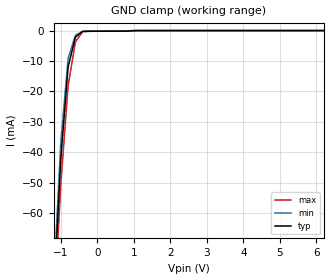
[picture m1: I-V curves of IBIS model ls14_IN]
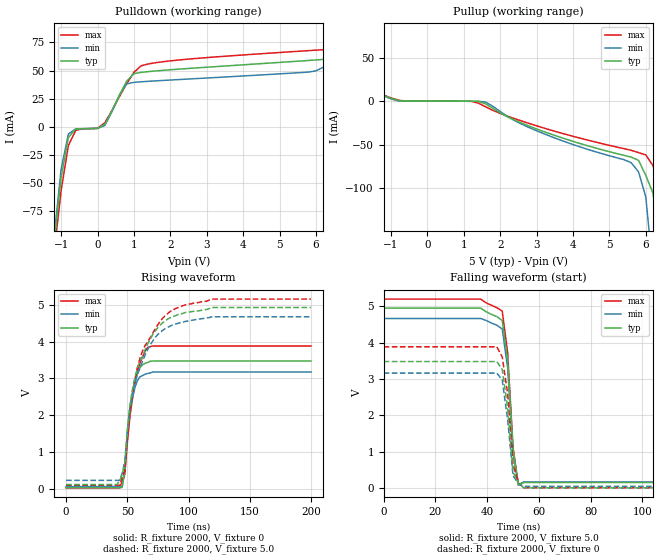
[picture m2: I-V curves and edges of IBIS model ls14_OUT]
|   TEXAS INSTRUMENTS INCORPORATED
|   Standard Linear and Logic Group
|   IBIS Model of SN74LS14
|   HEX SCHMITT- TRIGGER INVERTERS
|   SOIC 14-pin (D), SSOP 14-pin (DB),PDIP 14-pin (N)
[IBIS Ver]   3.2
[Comment Char]  |_char
[File Name]   sn74ls14.ibs
[File Rev]   3.2 | a_die
[Date]   11/12/04
[Source]   File originated at Texas Instruments, Inc.
[Notes]   The following is a sample IBIS file for the LS14.
   - FILE REV HISTORY
   - 3.2 Re-Release IBIS file on 11/16/04
   - Power clamp data deleted as there is no power-clamp diode.
   - All test data contained in this file are derived from
   actual measurement.
   - The measurement used NS package.
   - We have data across voltage and temperature, but not
   across process.
   - File created by Nobuhisa Ohtsubo, SLL Product Engineering.
[Disclaimer] Property of Texas Instruments Incorporated.  Unauthorized
   reproduction and/or distribution is strictly prohibited.
   This product is protected under copyright law.
   Created 2000, (C) Copyright 2000, Texas Instruments Inc.,
   All Rights Reserved.
   UNLESS THERE IS A SIGNED, WRITTEN AGREEMENT TO THE
   CONTRARY, TEXAS INSTRUMENTS () IS PROVIDING THE IBIS
   MODELS  AND WITHOUT ANY WARRANTY, EXPRESSED OR
   IMPLIED.  TI assumes no liability for:
   1) the accuracy of the IBIS models provided to your
   company;
   2) the proper functioning of these IBIS Models in your
   design or for any resulting applications; or
   3) infringement of patents, copyrights or intellectual
   property rights resulting from your use of these IBIS
   models.
   TI provides IBIS Models as a service to our customers.
   You and your company shall not distribute, sell or give
   these models to anyone else without prior written
   permission from TI.
   TI reserves the right to make changes to our products or
   to discontinue any semiconductor product or service
   without notice, and advises our customers to obtain the
   latest version of relevant information to verify, before
   placing orders, that the information being relied on is
   current.
   Please be aware that your receipt and use of the IBIS
   information provided shall serve as acceptance of these
   terms and conditions.  If you do not accept these terms,
   you should return or destroy the IBIS models and any
   other accompanying information immediately.
|   Component ls14_D
[Component]   ls14_D
[Manufacturer]  Texas Instruments, Inc.
[Package]
|   typ   min   max
R_pkg   0.031   0.028   0.034
L_pkg   3.109nH   2.462nH   3.889nH
C_pkg   0.473pF   0.363pF   0.628pF
[Pin]   signal_name   model_name   R_pin   L_pin   C_pin
1   1A   ls14_IN   0.033   3.854nH   0.622pF
2   1Y   ls14_OUT   0.032   3.188nH   0.473pF
3   2A   ls14_IN   0.028   2.462nH   0.377pF
4   2Y   ls14_OUT   0.031   2.596nH   0.363pF
5   3A   ls14_IN   0.028   2.521nH   0.372pF
6   3Y   ls14_OUT   0.034   3.250nH   0.476pF
7   GND   GND   0.034   3.889nH   0.628pF
8   4Y   ls14_IN   0.034   3.889nH   0.628pF
9   4A   ls14_OUT   0.034   3.250nH   0.476pF
10   5Y   ls14_IN   0.028   2.521nH   0.372pF
11   5A   ls14_OUT   0.031   2.596nH   0.364pF
12   6Y   ls14_IN   0.028   2.462nH   0.377pF
13   6A   ls14_OUT   0.032   3.188nH   0.473pF
14   VCC   POWER   0.033   3.854nH   0.622pF
| Component ls14_NS 14-pin SOP
[Component]   ls14_NS
[Manufacturer]   Texas Instruments, Inc.
[Package]
|   typ   min   max
R_pkg   0.045   0.039   0.054
L_pkg   3.796nH   2.561nH   4.952nH
C_pkg   0.528pF   0.288pF   0.710pF
[Pin]   signal_name   model_name   R_pin   L_pin   C_pin
1   1A   ls14_IN   0.047   4.867nH   0.706pF
2   1Y   ls14_OUT   0.051   4.083nH   0.592pF
3   2A   ls14_IN   0.041   2.915nH   0.376pF
4   2Y   ls14_OUT   0.039   2.561nH   0.288pF
5   3A   ls14_IN   0.041   3.101nH   0.430pF
6   3Y   ls14_OUT   0.047   4.047nH   0.589pF
7   GND   GND   0.051   4.909nH   0.700pF
8   4Y   ls14_IN   0.045   4.784nH   0.694pF
9   4A   ls14_OUT   0.054   4.176nH   0.597pF
10   5Y   ls14_IN   0.039   3.287nH   0.449pF
11   5A   ls14_OUT   0.039   2.586nH   0.294pF
12   6Y   ls14_IN   0.040   2.802nH   0.371pF
13   6A   ls14_OUT   0.049   4.080nH   0.593pF
14   VCC   POWER   0.052   4.952nH   0.710pF
| Component ls14_N 14-pin PDIP
[Component]   ls14_N
[Manufacturer]   Texas Instruments, Inc.
[Package]
|   typ   min   max
R_pkg   4.500e-02   3.700e-02   6.300e-02
L_pkg   5.407e-09   3.922e-09   6.942e-09
C_pkg   3.890e-13   2.050e-13   6.040e-13
[Pin]   signal_name   model_name   R_pin   L_pin   C_pin
1   1A   ls14_IN   6.300e-02   6.942e-09   6.040e-13
2   1Y   ls14_OUT   3.700e-02   6.200e-09   4.060e-13
3   2A   ls14_IN   4.200e-02   4.389e-09   3.220e-13
4   2Y   ls14_OUT   3.800e-02   3.922e-09   2.050e-13
5   3A   ls14_IN   3.900e-02   4.301e-09   2.980e-13
6   3Y   ls14_OUT   3.800e-02   5.329e-09   3.560e-13
7   GND   GND   5.300e-02   6.510e-09   5.440e-13
8   4Y   ls14_OUT   5.300e-02   6.437e-09   5.390e-13
9   4A   ls14_IN   3.900e-02   5.352e-09   3.470e-13
10   5Y   ls14_OUT   4.200e-02   4.473e-09   2.970e-13
11   5A   ls14_IN   4.400e-02   4.326e-09   2.250e-13
12   6Y   ls14_OUT   4.200e-02   4.295e-09   2.800e-13
13   6A   ls14_IN   4.200e-02   6.318e-09   4.180e-13
14   VCC   POWER   6.100e-02   6.900e-09   6.030e-13
|   Component ls14_DB
[Component]   ls14_DB
[Manufacturer]  Texas Instruments, Inc.
[Package]
|   typ   min   max
R_pkg   0.044   0.041   0.046
L_pkg   3.551nH   3.258nH   3.927nH
C_pkg   0.402pF   0.360pF   0.421pF
[Pin]   signal_name   model_name   R_pin   L_pin   C_pin
1   1A   ls14_IN   0.046   3.927nH   0.408pF
2   1Y   ls14_OUT   0.044   3.587nH   0.421pF
3   2A   ls14_IN   0.041   3.289nH   0.398pF
4   2Y   ls14_OUT   0.042   3.258nH   0.360pF
5   3A   ls14_IN   0.041   3.286nH   0.403pF
6   3Y   ls14_OUT   0.044   3.586nH   0.421pF
7   GND   GND   0.046   3.927nH   0.408pF
8   4Y   ls14_IN   0.046   3.927nH   0.408pF
9   4A   ls14_OUT   0.044   3.586nH   0.421pF
10   5Y   ls14_IN   0.041   3.286nH   0.403pF
11   5A   ls14_OUT   0.043   3.258nH   0.360pF
12   6Y   ls14_IN   0.041   3.289nH   0.398pF
13   6A   ls14_OUT   0.044   3.587nH   0.421pF
14   VCC   POWER   0.046   3.927nH   0.408pF
| Models and submodels in the file (2): ls14_IN (Input), ls14_OUT (Output)
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|   Model ls14_IN
[Model]   ls14_IN
Model_type  Input
Polarity   Inverting
Vinl = 0.8
Vinh = 2.0
| variable   typ   min   max
C_comp   1.33pf   1.00pf   1.66pf
[Temperature Range]   25   0   70
[Voltage Range]   5.0   4.75   5.25
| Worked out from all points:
|   GND clamp passes 1 mA (typ) near -0.48 V on its own axis
[GND Clamp]
|   Voltage   I(typ)   I(min)   I(max)
-5V       -1.315A    -1.382A    -1.195A
-1.2V     -88.77mA   -83.57mA   -95.34mA
-1V       -42.05mA   -36.6mA    -50.6mA
-800mV    -11.89mA   -9.112mA   -18.14mA
-600mV    -2.169mA   -1.53mA    -3.706mA
-400mV    -247.6uA   -246.4uA   -364uA
1.2V      -366.4nA   -227.1nA   -428nA
10V       15.2nA     25.25nA    57.62nA
|   Model ls14_OUT
[Model]   ls14_OUT
Model_type  Output
Polarity   Inverting
Vmeas = 1.3v
Cref = 15pf
Rref = 2000
Vref = 0V
| variable   typ   min   max
C_comp   5.8pf   4.35pf   7.25pf
[Temperature Range]   25   0   70
[Voltage Range]   5.0   4.75   5.25
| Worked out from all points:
|   slope of the pulldown table from 0 to 0.75 V, typ, clamps not added: 19.3 ohm
|   slope of the pullup table from 0 to 0.75 V, typ, clamps not added: 31.3 kohm
|   rising waveform, R_fixture 2000, V_fixture 0: 20-80 % time 7.12ns typ, 6.52ns min, 8.96ns max; typ from 0.022 V to 3.47 V
|   falling waveform, R_fixture 2000, V_fixture 5.0: 20-80 % time 2.91ns typ, 2.91ns min, 2.89ns max; typ from 4.95 V to 0.156 V
|   rising waveform, R_fixture 2000, V_fixture 5.0: 20-80 % time 18.3ns typ, 17.7ns min, 19.9ns max; typ from 0.11 V to 4.93 V
|   falling waveform, R_fixture 2000, V_fixture 0: 20-80 % time 2.93ns typ, 2.89ns min, 3.01ns max; typ from 3.48 V to 0.011 V
[Pulldown]
|   Voltage   I(typ)   I(min)   I(max)
-5V       -1.637A    -1.754A    -1.459A
-1.2V     -106.1mA   -99.87mA   -113.9mA
-1V       -45.11mA   -37.62mA   -56.62mA
-800mV    -9.35mA    -6.287mA   -16.52mA
-600mV    -1.967mA   -1.716mA   -3.114mA
200mV     2.325mA    1.242mA    3.681mA
800mV     40.65mA    38.22mA    38.31mA
1.2V      48.39mA    40.06mA    54.31mA
6V        59.43mA    49.77mA    68.14mA
6.6V      64.1mA     61.17mA    69.39mA
7.8V      87.38mA    87.2mA     82.72mA
10V       130.7mA    135.2mA    111.3mA
[Pullup]
|   Voltage   I(typ)   I(min)   I(max)
-5V       79.98mA    83.78mA    71.9mA
-1V       3.053mA    2.551mA    3.692mA
1.2V      -122.7uA   -120.8uA   -176.8uA
1.6V      -3.112mA   -1.033mA   -6.444mA
3V        -31.9mA    -33.98mA   -28.32mA
5.6V      -64.26mA   -70.72mA   -56.46mA
5.8V      -67.99mA   -81.16mA   -59.07mA
6V        -85.2mA    -110mA     -61.78mA
6.2V      -106mA     -197.1mA   -74.27mA
6.4V      -178.6mA   -282.8mA   -98.07mA
6.6V      -257.9mA   -372.3mA   -162.3mA
10V       -1.647A    -1.884A    -1.38A
[Ramp]
| variable   typ   min   max
dV/dt_r  2.028E+00/1.033E-08  1.854E-01/1.005E-08  2.256E+00/1.186E-08
dV/dt_f  2.920E+00/1.781E-09  2.766E+00/2.766E-09  3.084E+00/1.656E-09
R_load = 2000
[Rising Waveform]
R_fixture = 2000
V_fixture = 0
V_fixture_min = 0
V_fixture_max = 0
C_fixture = 0pf
L_fixture = 0nH
|   Time   V(typ)   V(min)   V(max)
0s        21.98mV    53.41mV    20.04mV
43.75ns   22.44mV    54.19mV    20.18mV
45.83ns   32.5mV     56.19mV    189.7mV
47.92ns   507.3mV    483.6mV    378.3mV
50ns      1.494V     1.469V     1.233V
52.08ns   2.151V     2.099V     1.945V
56.25ns   2.906V     2.754V     2.858V
60.42ns   3.302V     3.047V     3.419V
66.67ns   3.437V     3.136V     3.844V
200ns     3.474V     3.176V     3.883V
[Falling Waveform]
R_fixture = 2000
V_fixture = 5.0
V_fixture_min = 4.75
V_fixture_max = 5.25
C_fixture = 0pf
L_fixture = 0nH
|   Time   V(typ)   V(min)   V(max)
0s        4.951V     4.666V     5.198V
37.5ns    4.951V     4.666V     5.198V
39.58ns   4.853V     4.612V     5.096V
43.75ns   4.717V     4.481V     4.963V
45.83ns   4.612V     4.377V     4.868V
47.92ns   3.541V     3.309V     3.73V
50ns      1.058V     992.8mV    1.131V
52.08ns   83.54mV    86.14mV    108.1mV
54.17ns   156mV      172.4mV    166.7mV
200ns     156mV      172.4mV    166.7mV
[Rising Waveform]
R_fixture = 2000
V_fixture = 5.0
V_fixture_min = 4.75
V_fixture_max = 5.25
C_fixture = 0pf
L_fixture = 0nH
|   Time   V(typ)   V(min)   V(max)
0s        110.1mV    223.9mV    89mV
43.75ns   223.4mV    228.2mV    89.85mV
47.92ns   676.2mV    731.1mV    483.5mV
52.08ns   2.26V      2.217V     2.067V
56.25ns   3.031V     2.886V     2.983V
60.42ns   3.471V     3.287V     3.557V
72.92ns   4.296V     4.122V     4.358V
85.42ns   4.659V     4.433V     4.834V
118.8ns   4.931V     4.679V     5.16V
200ns     4.931V     4.679V     5.16V
[Falling Waveform]
R_fixture = 2000
V_fixture = 0
V_fixture_min = 0
V_fixture_max = 0
C_fixture = 0pf
L_fixture = 0nH
|   Time   V(typ)   V(min)   V(max)
0s        3.482V     3.165V     3.889V
43.75ns   3.482V     3.165V     3.889V
45.83ns   3.265V     2.978V     3.609V
47.92ns   2.207V     1.891V     2.605V
50ns      451.3mV    348.9mV    663.8mV
52.08ns   125.5mV    120.8mV    139.2mV
54.17ns   12.31mV    52.58mV    14.21mV
56.25ns   11.04mV    52.44mV    13.22mV
200ns     11.04mV    52.44mV    13.22mV
